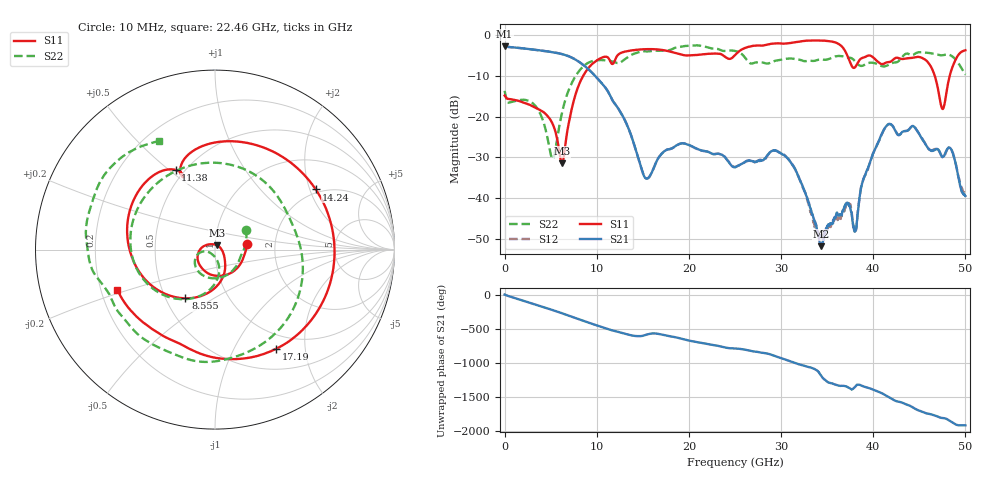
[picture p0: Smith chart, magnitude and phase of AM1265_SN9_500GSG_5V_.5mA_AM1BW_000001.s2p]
!Keysight Technologies,N5245B,MY58422270,A.16.20.02
!Date: Thursday, March 05, 2026 00:25:28
!Correction: S11(C  2-Port  )
!S21(C  2-Port  )
!S12(C  2-Port  )
!S22(C  2-Port  )
!S2P File: Measurements: S11, S21, S12, S22:
# Hz S  dB  R 50
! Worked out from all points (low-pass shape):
!   3201 points, 10 MHz to 50 GHz, reference 50 ohm
!   highest |S21| = -2.82 dB at 10 MHz (marker M1); lowest = -51.7 dB at 34.35 GHz (marker M2)
!   |S21| within 3 dB of the highest: start of sweep to 7.502 GHz
!   lowest |S11| = -31.4 dB at 6.228 GHz (marker M3), VSWR 1.06, Z = 51 + j2.52 ohm
!   |S11| at or under -10 dB: start of sweep to 8.547 GHz; 46.67 GHz to 48.3 GHz (1.631 GHz wide, 3.43 % of centre)
!   |S22| runs from -30.3 to -2.6 dB; largest |S21 - S12| = 0.0094
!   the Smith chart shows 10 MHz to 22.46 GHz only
!   S11 on the Smith chart (normalised r, x): 10 MHz: 1.43, +0.09; 8.555 GHz: 0.63, -0.38; 11.38 GHz: 0.45, +0.53; 14.24 GHz: 1.88, +2.20; 17.19 GHz: 0.78, -1.49; 22.46 GHz: 0.27, -0.18
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1e7  -14.86 9.9  -2.82 3.8  -2.86 3.1  -13.71 32.7
1.931491e9  -16.48 -77.1  -3.30 -82.5  -3.31 -82.5  -15.89 -96.0
3.852981e9  -18.39 -136.3  -3.81 -164.2  -3.82 -164.1  -19.21 -160.5
5.212084e9  -21.76 178.2  -4.26 136.2  -4.26 136.3  -30.35 -128.8
6.227506e9  -31.40 66.3  -4.71 89.7  -4.72 89.7  -19.18 -77.5
8.352081e9  -10.83 -112.0  -7.05 -11.9  -7.04 -11.8  -8.16 -141.5
8.555166e9  -9.97 -121.2  -7.40 -21.5  -7.39 -21.4  -7.70 -149.2
1.138272e10  -6.10 116.3  -14.55 -150.4  -14.55 -150.4  -6.36 80.5
1.424153e10  -3.69 30.8  -28.16 115.7  -28.22 115.8  -4.49 -70.2
1.667854e10  -3.59 -44.2  -30.18 147.1  -30.19 147.3  -3.94 -140.9
1.719406e10  -3.75 -58.3  -28.75 133.6  -28.80 133.4  -3.86 -150.7
2.245863e10  -4.61 -157.7  -29.03 -12.7  -29.07 -12.4  -3.34 117.1
2.5005e10  -4.97 174.9  -32.40 -66.4  -32.34 -66.6  -3.96 70.9
3.023833e10  -2.17 85.0  -29.35 140.7  -29.17 141.1  -5.99 -41.0
3.334708e10  -1.41 35.6  -43.60 5.8  -43.92 3.2  -6.39 -126.5
3.434688e10  -1.39 18.2  -51.71 -105.6  -49.31 -92.2  -6.04 -147.4
3.672141e10  -3.18 -31.9  -42.93 105.4  -43.53 108.5  -5.28 165.9
3.804927e10  -7.90 -25.5  -48.01 93.1  -48.35 -179.8  -6.53 139.7
4.167354e10  -6.68 -53.5  -21.83 -59.9  -21.85 -59.4  -7.34 117.0
4.511035e10  -5.50 -100.9  -24.74 93.6  -24.67 94.3  -4.23 75.6
4.770358e10  -17.27 68.2  -29.58 -9.0  -29.78 -7.8  -4.93 39.7
5e10  -3.79 -71.3  -39.45 -114.9  -38.29 -122.0  -9.73 2.5
